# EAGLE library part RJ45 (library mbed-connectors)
Magjack SI-68002
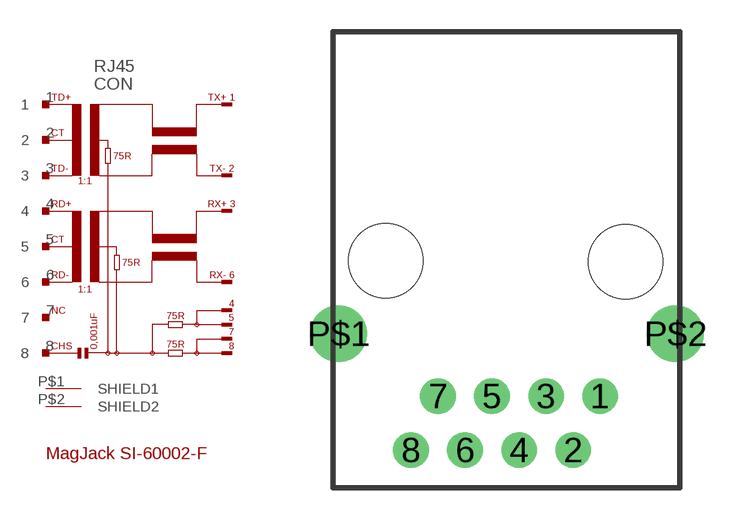
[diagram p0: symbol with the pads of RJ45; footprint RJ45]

Designator prefix CON

## RJ45  [RJ45]
1  1  pas
2  2  pas
3  3  pas
4  4  pas
5  5  pas
6  6  pas
7  7  pas
8  8  pas
P$1  SHIELD1
P$2  SHIELD2

## Footprint RJ45 (pad centres in mm)
drill 1.016 pad 1.676: 1 0,0; 2 -1.27,-2.54; 3 -2.54,0; 4 -3.81,-2.54; 5 -5.08,0; 6 -6.35,-2.54; 7 -7.62,0; 8 -8.89,-2.54
drill 1.778: P$1 -12.3,2.95; P$2 3.55,2.95
hole 3.5 at -10.09,6.38
hole 3.5 at 1.21,6.33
